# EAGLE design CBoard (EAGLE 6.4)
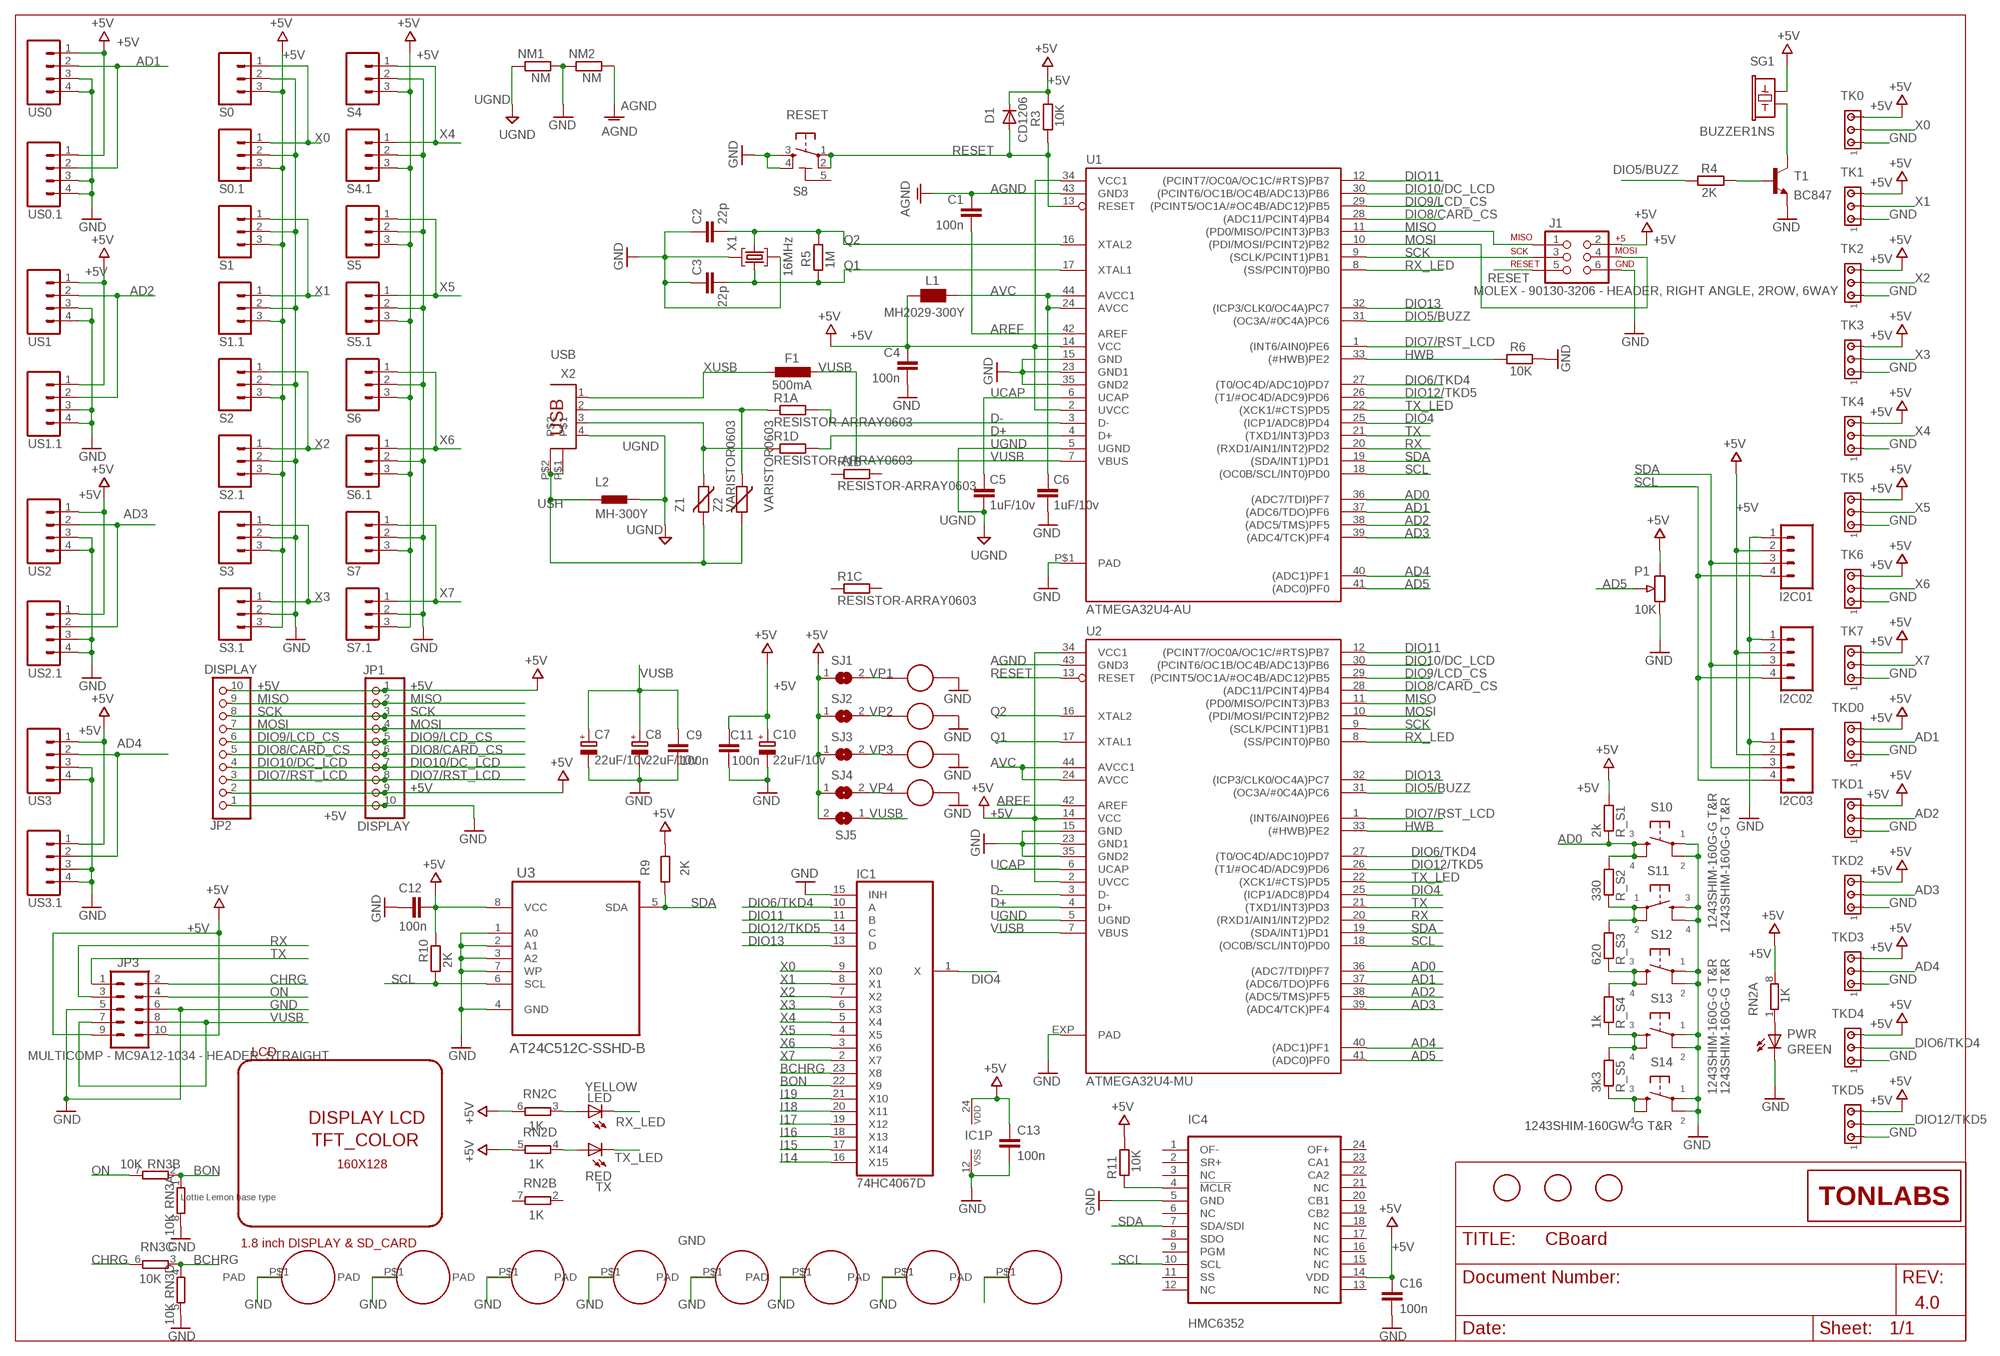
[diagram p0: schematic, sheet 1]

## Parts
1  FIDUCIALMOUNT  [FIDUCIA-MOUNT]
2  FIDUCIALMOUNT  [FIDUCIA-MOUNT]
3  FIDUCIALMOUNT  [FIDUCIA-MOUNT]
C1  100n  C-EUC0603  [C0603-ROUND]
C2  22p  C-EUC0603  [C0603-ROUND]
C3  22p  C-EUC0603  [C0603-ROUND]
C4  100n  C-EUC0603  [C0603-ROUND]
C5  1uF/10v  C-EUC0603  [C0603-ROUND]
C6  1uF/10v  C-EUC0603  [C0603-ROUND]
C7  22uF/10v  CPOL-EUSMCB  [SMC_B]
C8  22uF/10v  CPOL-EUSMCB  [SMC_B]
C9  100n  C-EUC0603  [C0603-ROUND]
C10  22uF/10v  CPOL-EUSMCB  [SMC_B]
C11  100n  C-EUC0603  [C0603-ROUND]
C12  100n  C-EUC0603  [C0603-ROUND]
C13  100n  C-EUC0603  [C0603-ROUND]
C16  100n  C-EUC0603  [C0603-ROUND]
D1  CD1206  DIODE-MINIMELF  [MINIMELF]
F1  500mA  L-EUL1812  [L1812]
G1  LOTTIE_LEMON_BASE_TYPE  [BASE_ROBOT_001]
H1  2.5-MOUNTING-HOLE  [2.5PAD]
H2  2.5-MOUNTING-HOLE  [2.5PAD]
H3  2.5-MOUNTING-HOLE  [2.5PAD]
H4  2.5-MOUNTING-HOLE  [2.5PAD]
H5  2.5-MOUNTING-HOLE  [2.5PAD]
H6  2.5-MOUNTING-HOLE  [2.5PAD]
H7  2.5-MOUNTING-HOLE  [2.5PAD]
H8  2.5-MOUNTING-HOLE  [2.5PAD]
I2C01  M04PTH  [1X04]
I2C02  M04PTH  [1X04]
I2C03  M04PTH  [1X04]
IC1  74HC4067D  4067D  [SO24W]
IC4  HMC6352  [HMC6352]
J1  MOLEX - 90130-3206 - HEADER, RIGHT ANGLE, 2ROW, 6WAY  AVR_SPI_PRG_6PTH  [2X3]
JP1  DISPLAY  PINHD-1X10TH  [1X10-TH]
JP2  DISPLAY  PINHD-1X10TH  [1X10-TH]
JP3  MULTICOMP - MC9A12-1034 - HEADER, STRAIGHT  M05X2SHD_LOCK  [2X5-SHROUDED_LOCK]
L1  MH2029-300Y  WE-CBF_0805  [0805]
L2  MH-300Y  BEAD0805  [BEAD-0805-SMT]
LCD  1.8 inch DISPLAY & SD_CARD  1.8-COLOR_TFT-LCD_DISPLAY_&_MICRO-SD  [1.8-LCD]
LED  YELLOW  LEDCHIP-LED0805  [CHIP-LED0805]
LOGO  LOGO-TONYLABSMED-LANDSCAPE  [LOGO-TONYLABS-MED-LANDSCAPE]
NM1  NM  R-EU_R0805  [R0805]
NM2  NM  R-EU_R0805  [R0805]
P1  10K  POT-VERTICAL  [POT-V]
PTZ1  LOTTIE_LEMON_PADS_SUP  [PADS_LOTTIE_LEMON_SUP]
PTZ2  LOTTIE_LEMON_PADS_SUP  [PADS_LOTTIE_LEMON_SUP]
PTZ3  LOTTIE_LEMON_PADS_SUP1  [PADS_LOTTIE_LEMON_SUP]
PTZ4  LOTTIE_LEMON_PADS_SUP1  [PADS_LOTTIE_LEMON_SUP]
PWR  LEDCHIP-LED0805  [CHIP-LED0805]
R1  RESISTOR-ARRAY0603  [RESISTOR-0603-SMT-ARRAY]
R3  10K  R-EU_R0603  [R0603-ROUND]
R4  2K  R-EU_R0603  [R0603-ROUND]
R5  1M  R-EU_R0603  [R0603-ROUND]
R6  10K  R-EU_R0603  [R0603-ROUND]
R9  2K  R-EU_R0603  [R0603-ROUND]
R10  2K  R-EU_R0603  [R0603-ROUND]
R11  10K  R-EU_R0603  [R0603-ROUND]
R_S1  2k  R-EU_R0603  [R0603-ROUND]
R_S2  330  R-EU_R0603  [R0603-ROUND]
R_S3  620  R-EU_R0603  [R0603-ROUND]
R_S4  1k  R-EU_R0603  [R0603-ROUND]
R_S5  3k3  R-EU_R0603  [R0603-ROUND]
RN2  1K  4R-NCAY16  [CAY16]
RN3  10K  4R-NCAY16  [CAY16]
S0  M03PTH  [1X03]
S0.1  M03PTH  [1X03]
S1  M03PTH  [1X03]
S1.1  M03PTH  [1X03]
S2  M03PTH  [1X03]
S2.1  M03PTH  [1X03]
S3  M03PTH  [1X03]
S3.1  M03PTH  [1X03]
S4  M03PTH  [1X03]
S4.1  M03PTH  [1X03]
S5  M03PTH  [1X03]
S5.1  M03PTH  [1X03]
S6  M03PTH  [1X03]
S6.1  M03PTH  [1X03]
S7  M03PTH  [1X03]
S7.1  M03PTH  [1X03]
S8  RESET  TS42  [TS42]
S10  1243SHIM-160G-G T&R  TACTILE_SWITCHTACTILE_SWITCH_SMD-12MM  [TACTILE-SMD-12MM]
S11  1243SHIM-160G-G T&R  TACTILE_SWITCHTACTILE_SWITCH_SMD-12MM  [TACTILE-SMD-12MM]
S12  1243SHIM-160G-G T&R  TACTILE_SWITCHTACTILE_SWITCH_SMD-12MM  [TACTILE-SMD-12MM]
S13  1243SHIM-160G-G T&R  TACTILE_SWITCHTACTILE_SWITCH_SMD-12MM  [TACTILE-SMD-12MM]
S14  1243SHIM-160GW-G T&R  TACTILE_SWITCHTACTILE_SWITCH_SMD-12MM  [TACTILE-SMD-12MM]
SG1  BUZZER1NS  [BUZZER-12MM-NS]
SJ1  SJ  [SJ]
SJ2  SJ  [SJ]
SJ3  SJ  [SJ]
SJ4  SJ  [SJ]
SJ5  SJL  [SJL]
T1  BC847  [SOT23]
TK0  MTA03-100  [10X03MTA]
TK1  MTA03-100  [10X03MTA]
TK2  MTA03-100  [10X03MTA]
TK3  MTA03-100  [10X03MTA]
TK4  MTA03-100  [10X03MTA]
TK5  MTA03-100  [10X03MTA]
TK6  MTA03-100  [10X03MTA]
TK7  MTA03-100  [10X03MTA]
TKD0  MTA03-100  [10X03MTA]
TKD1  MTA03-100  [10X03MTA]
TKD2  MTA03-100  [10X03MTA]
TKD3  MTA03-100  [10X03MTA]
TKD4  MTA03-100  [10X03MTA]
TKD5  MTA03-100  [10X03MTA]
TX  RED  LEDCHIP-LED0805  [CHIP-LED0805]
U1  ATMEGA32U4-AU  ATMEGA32U4-XUAU  [TQFP44-PAD]
U2  ATMEGA32U4-MU  ATMEGA32U4-XUMU  [QFN44ML7X7]
U3  AT24C512C-SSHD-B  AT24C128BN-SH-B  [SOIC127P600X175-8N]
US0  M04PTH  [1X04]
US0.1  M04PTH  [1X04]
US1  M04PTH  [1X04]
US1.1  M04PTH  [1X04]
US2  M04PTH  [1X04]
US2.1  M04PTH  [1X04]
US3  M04PTH  [1X04]
US3.1  M04PTH  [1X04]
X1  16MHz  CRYSTAL-3.2-2.5  [CRYSTAL-3.2-2.5]
X2  USB  PN61729  [PN61729]
Z1  VARISTOR0603  [VARISTOR-0603-SMT]
Z2  VARISTOR0603  [VARISTOR-0603-SMT]

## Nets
+5V: C4.1 C10.+ C11.1 C12.1 C13.1 C16.1 D1.C I2C01.2 I2C02.2 I2C03.2 IC1.24(VDD) IC4.14(VDD) J1.2 JP1.1 JP1.9 JP2.2 JP2.10 JP3.9 JP3.10 L1.2 P1.B R3.1 R9.2 R10.1 R11.1 R_S1.2 RN2.5 RN2.6 RN2.8 S0.1.3 S0.3 S1.1.3 S1.3 S2.1.3 S2.3 S3.1.3 S3.3 S4.1.3 S4.3 S5.1.3 S5.3 S6.1.3 S6.3 S7.1.3 S7.3 SG1.+ SJ1.1 SJ2.1 SJ3.1 SJ4.1 SJ5.2 TK0.3 TK1.3 TK2.3 TK3.3 TK4.3 TK5.3 TK6.3 TK7.3 TKD0.3 TKD1.3 TKD2.3 TKD3.3 TKD4.3 TKD5.3 U1.2(UVCC) U1.14(VCC) U1.34(VCC1) U2.2(UVCC) U2.14(VCC) U2.34(VCC1) U3.8(VCC) US0.1 US0.1.1 US1.1 US1.1.1 US2.1 US2.1.1 US3.1 US3.1.1
AD0: R_S1.1 R_S2.2 S10.P$3 S10.P$4 U1.36((ADC7/TDI)PF7) U2.36((ADC7/TDI)PF7)
AD1: TKD0.2 U1.37((ADC6/TDO)PF6) U2.37((ADC6/TDO)PF6) US0.1.2 US0.2
AD2: TKD1.2 U1.38((ADC5/TMS)PF5) U2.38((ADC5/TMS)PF5) US1.1.2 US1.2
AD3: TKD2.2 U1.39((ADC4/TCK)PF4) U2.39((ADC4/TCK)PF4) US2.1.2 US2.2
AD4: TKD3.2 U1.40((ADC1)PF1) U2.40((ADC1)PF1) US3.1.2 US3.2
AD5: P1.C U1.41((ADC0)PF0) U2.41((ADC0)PF0)
AGND: C1.1 NM2.1 U1.43(GND3) U2.43(GND3)
AREF: C1.2 U1.42(AREF) U2.42(AREF)
AVC: C6.1 L1.1 U1.24(AVCC) U1.44(AVCC1) U2.24(AVCC) U2.44(AVCC1)
BCHRG: IC1.23(X8) RN3.3 RN3.4
BON: IC1.22(X9) RN3.1 RN3.2
CHRG: JP3.2 RN3.6
D+: R1.5 U1.4(D+) U2.4(D+)
D-: R1.8 U1.3(D-) U2.3(D-)
DIO4: IC1.1(X) U1.25((ICP1/ADC8)PD4) U2.25((ICP1/ADC8)PD4)
DIO5/BUZZ: R4.2 U1.31((OC3A/#0C4A)PC6) U2.31((OC3A/#0C4A)PC6)
DIO6/TKD4: IC1.10(A) TKD4.2 U1.27((T0/OC4D/ADC10)PD7) U2.27((T0/OC4D/ADC10)PD7)
DIO7/RST_LCD: JP1.8 JP2.3 U1.1((INT6/AIN0)PE6) U2.1((INT6/AIN0)PE6)
DIO8/CARD_CS: JP1.6 JP2.5 U1.28((ADC11/PCINT4)PB4) U2.28((ADC11/PCINT4)PB4)
DIO9/LCD_CS: JP1.5 JP2.6 U1.29((PCINT5/OC1A/#OC4B/ADC12)PB5) U2.29((PCINT5/OC1A/#OC4B/ADC12)PB5)
DIO10/DC_LCD: JP1.7 JP2.4 U1.30((PCINT6/OC1B/OC4B/ADC13)PB6) U2.30((PCINT6/OC1B/OC4B/ADC13)PB6)
DIO11: IC1.11(B) U1.12((PCINT7/OC0A/OC1C/#RTS)PB7) U2.12((PCINT7/OC0A/OC1C/#RTS)PB7)
DIO12/TKD5: IC1.14(C) TKD5.2 U1.26((T1/#OC4D/ADC9)PD6) U2.26((T1/#OC4D/ADC9)PD6)
DIO13: IC1.13(D) U1.32((ICP3/CLK0/OC4A)PC7) U2.32((ICP3/CLK0/OC4A)PC7)
GND: C2.1 C3.1 C4.2 C6.2 C7.- C8.- C9.2 C10.- C11.2 C12.2 C13.2 C16.2 H1.P$1(PAD) H2.P$1(PAD) H3.P$1(PAD) H4.P$1(PAD) H5.P$1(PAD) H6.P$1(PAD) H7.P$1(PAD) H8.P$1(PAD) I2C01.1 I2C02.1 I2C03.1 IC1.12(VSS) IC1.15(INH) IC4.5(GND) J1.6 JP1.10 JP2.1 JP3.5 JP3.6 NM1.1 NM2.2 P1.A PTZ1.P$52 PTZ2.P$52 PTZ3.P$52 PTZ4.P$52 PWR.C R6.1 RN3.5 RN3.8 S0.1.2 S0.2 S1.1.2 S1.2 S2.1.2 S2.2 S3.1.2 S3.2 S4.1.2 S4.2 S5.1.2 S5.2 S6.1.2 S6.2 S7.1.2 S7.2 S8.3 S8.4 S10.P$1 S10.P$2 S11.P$3 S11.P$4 S12.P$1 S12.P$2 S13.P$1 S13.P$2 S14.P$1 S14.P$2 T1.2(E) TK0.1 TK1.1 TK2.1 TK3.1 TK4.1 TK5.1 TK6.1 TK7.1 TKD0.1 TKD1.1 TKD2.1 TKD3.1 TKD4.1 TKD5.1 U1.15(GND) U1.23(GND1) U1.35(GND2) U1.P$1(PAD) U2.15(GND) U2.23(GND1) U2.35(GND2) U2.EXP(PAD) U3.1(A0) U3.2(A1) U3.3(A2) U3.4(GND) U3.7(WP) US0.1.3 US0.1.4 US0.3 US0.4 US1.1.3 US1.1.4 US1.3 US1.4 US2.1.3 US2.1.4 US2.3 US2.4 US3.1.3 US3.1.4 US3.3 US3.4 X1.2(GND) X1.4(GND)
HWB: R6.2 U1.33((#HWB)PE2) U2.33((#HWB)PE2)
I14: IC1.16(X15)
I15: IC1.17(X14)
I16: IC1.18(X13)
I17: IC1.19(X12)
I18: IC1.20(X11)
I19: IC1.21(X10)
MISO: J1.1 JP1.2 JP2.9 U1.11((PD0/MISO/PCINT3)PB3) U2.11((PD0/MISO/PCINT3)PB3)
MOSI: J1.4 JP1.4 JP2.7 U1.10((PDI/MOSI/PCINT2)PB2) U2.10((PDI/MOSI/PCINT2)PB2)
N$2: R1.1 X2.2 Z2.1
N$3: R1.4 X2.3 Z1.1
N$4: RN2.4 TX.A
N$5: IC4.4(!MCLR) R11.2
N$13: R_S2.1 R_S3.2 S11.P$1 S11.P$2
N$14: LED.A RN2.3
N$17: SG1.- T1.3(C)
N$24: PWR.A RN2.1
N$27: R_S3.1 R_S4.2 S12.P$3 S12.P$4
N$29: R_S4.1 R_S5.2 S13.P$3 S13.P$4
N$30: R_S5.1 S14.P$3 S14.P$4
N$31: R4.1 T1.1(B)
ON: JP3.4 RN3.7
Q1: C3.2 R5.2 U1.17(XTAL1) U2.17(XTAL1) X1.1(C1)
Q2: C2.2 R5.1 U1.16(XTAL2) U2.16(XTAL2) X1.3(C2)
RESET: D1.A J1.5 R3.2 S8.1 S8.2 U1.13(RESET) U2.13(RESET)
RX: JP3.3 U1.20((RXD1/AIN1/INT2)PD2) U2.20((RXD1/AIN1/INT2)PD2)
RX_LED: LED.C U1.8((SS/PCINT0)PB0) U2.8((SS/PCINT0)PB0)
SCK: J1.3 JP1.3 JP2.8 U1.9((SCLK/PCINT1)PB1) U2.9((SCLK/PCINT1)PB1)
SCL: I2C01.4 I2C02.4 I2C03.4 IC4.10(SCL) R10.2 U1.18((OC0B/SCL/INT0)PD0) U2.18((OC0B/SCL/INT0)PD0) U3.6(SCL)
SDA: I2C01.3 I2C02.3 I2C03.3 IC4.7(SDA/SDI) R9.1 U1.19((SDA/INT1)PD1) U2.19((SDA/INT1)PD1) U3.5(SDA)
TX: JP3.1 U1.21((TXD1/INT3)PD3) U2.21((TXD1/INT3)PD3)
TX_LED: TX.C U1.22((XCK1/#CTS)PD5) U2.22((XCK1/#CTS)PD5)
UCAP: C5.1 U1.6(UCAP) U2.6(UCAP)
UGND: C5.2 L2.2 NM1.2 U1.5(UGND) U2.5(UGND) X2.4
USH: L2.1 X2.P$1 X2.P$2 Z1.2 Z2.2
VP1: PTZ3.P$42 SJ1.2
VP2: PTZ4.P$42 SJ2.2
VP3: PTZ1.P$42 SJ3.2
VP4: PTZ2.P$42 SJ4.2
VUSB: C7.+ C8.+ C9.1 F1.2 JP3.7 JP3.8 SJ5.1 U1.7(VBUS) U2.7(VBUS)
X0: IC1.9(X0) S0.1 S0.1.1 TK0.2
X1: IC1.8(X1) S1.1 S1.1.1 TK1.2
X2: IC1.7(X2) S2.1 S2.1.1 TK2.2
X3: IC1.6(X3) S3.1 S3.1.1 TK3.2
X4: IC1.5(X4) S4.1 S4.1.1 TK4.2
X5: IC1.4(X5) S5.1 S5.1.1 TK5.2
X6: IC1.3(X6) S6.1 S6.1.1 TK6.2
X7: IC1.2(X7) S7.1 S7.1.1 TK7.2
XUSB: F1.1 X2.1
Unconnected: IC4.1(OF-) IC4.2(SR+) IC4.3(NC) IC4.6(NC) IC4.8(SDO) IC4.9(PGM) IC4.11(SS) IC4.12(NC) IC4.13(NC) IC4.15(NC) IC4.16(NC) IC4.17(NC) IC4.18(NC) IC4.19(CB2) IC4.20(CB1) IC4.21(NC) IC4.22(CA2) IC4.23(CA1) IC4.24(OF+) R1.2 R1.3 R1.6 R1.7 RN2.2 RN2.7

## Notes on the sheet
- GREEN
- 4.0

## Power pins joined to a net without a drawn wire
5-GND: S8.5(5-GND)

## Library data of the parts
1-3 = Smartprj:FIDUCIALMOUNT
C1-C6 C9 C11-C13 C16 = Smartprj:C-EU: CAPACITOR, European symbol
C7 C8 C10 = Smartprj:CPOL-EU: POLARIZED CAPACITOR, European symbol
D1 = diode:DIODE-: DIODE
F1 = rcl:L-EU: INDUCTOR, European symbol
G1 = complubot:LOTTIE_LEMON_BASE_TYPE: Lottie Lemon Robot Base
H1-H8 = tinker_it:2.5-MOUNTING-HOLE
I2C01-I2C03 US0 US0.1 US1 US1.1 US2 US2.1 US3 US3.1 = sparkfun:M04: Header 4 Standard 4-pin 0.1" header. Use with straight break away headers (SKU : PRT-00116), right angle break away headers (PRT-00553), swiss pins (PRT-00743), machine pins (PRT-00117), and female headers (PRT-00115). Molex polarized connector foot print use with SKU : PRT-08231 with associated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
IC1 = 40xx:4067: 16-channel ANALOG MULTIPLEXER
IC4 = Smartprj:HMC6352: HMC6352 2-Axis Compass with Algorithms Honeywell
J1 = sparkfun:AVR_SPI_PRG_6: AVR ISP 6 Pin This is the reduced ISP connector for AVR programming. Common on Arduino. This footprint will take up less PCB space and can be used with a 10-pin to 6-pin adapter such as SKU: BOB-08508
JP1 JP2 = Smartprj:PINHD-1X10: PIN HEADER
JP3 = Smartprj:M05X2: Header 5x2 Standard 10-pin dual row 0.1" header. Commonly used with AVR-ISP. Use with Spark Fun Electronics SKU: PRT-00778
L1 = wuerth-elektronik:WE-CBF: SMD EMI Suppression Ferrite Beads
L2 = TONYLABS:BEAD
LCD = Smartprj:1.8-COLOR_TFT-LCD_DISPLAY_&_MICRO-SD: 1.8 inch LCD_COLOR
LED PWR TX = led:LED: LED
LOGO = TONYLABS:LOGO-TONYLABS
NM1 NM2 = resistor:R-EU_: RESISTOR, European symbol
P1 = Smartprj:POT-VERTICAL: Vertical POT TinkerKit
PTZ1 PTZ2 = Lottie_SPad2:LOTTIE_LEMON_PADS_SUP
PTZ3 PTZ4 = Lottie_SPad:LOTTIE_LEMON_PADS_SUP1
R1 = TONYLABS:RESISTOR-ARRAY; PACKAGE: 0603
R3-R6 R9-R11 R_S1-R_S5 = Smartprj:R-EU_: RESISTOR, European symbol
RN2 RN3 = resistor-dil:4R-N: Array Chip Resistor Source: RS Component / Phycomp; OC_FARNELL: unknown; OC_NEWARK: unknown
S0 S0.1 S1 S1.1 S2 S2.1 S3 S3.1 S4 S4.1 S5 S5.1 S6 S6.1 S7 S7.1 = sparkfun:M03: Header 3 Standard 3-pin 0.1" header. Use with straight break away headers (SKU : PRT-00116), right angle break away headers (PRT-00553), swiss pins (PRT-00743), machine pins (PRT-00117), and female headers (PRT-00115). Molex polarized connector foot print use with SKU : PRT-08232 with associated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
S8 = Smartprj:TS42: TS42 Dongnan Electronics Tact switch VDC 12V - 50mA
S10-S14 = Smartprj:TACTILE_SWITCH: Momentary Switch Button commonly used for reset or general input.
SG1 = Smartprj:BUZZER1: Buzzer 12-22mm
SJ1-SJ5 = Smartprj:SJ: SMD solder JUMPER
T1 = transistor:BC847: NPN TRANSISTOR
TK0 TK1-TK7 TKD0 TKD1-TKD5 = con-amp:MTA03-100: AMP connector
U1 U2 = Smartprj:ATMEGA32U4-XU
U3 = Smartprj:AT24C128BN-SH-B: Two-wire Serial EEPROM; MPN: AT24C128BN-SH-B; OC_FARNELL: 1362649; OC_NEWARK: 50M3322; PACKAGE: SOIC-8; SUPPLIER: Atmel
X1 = Smartprj:CRYSTAL-3.2-2.5
X2 = Smartprj:PN61729: BERG USB connector
Z1 Z2 = TONYLABS:VARISTOR: Varistor

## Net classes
0 default: width 0.254 mm, drill 0.584 mm, clearance 0.178 mm
1 +5V: width 0.254 mm, drill 0.787 mm, clearance 0.178 mm
2 gnd: width 0.254 mm, drill 0.584 mm, clearance 0.178 mm

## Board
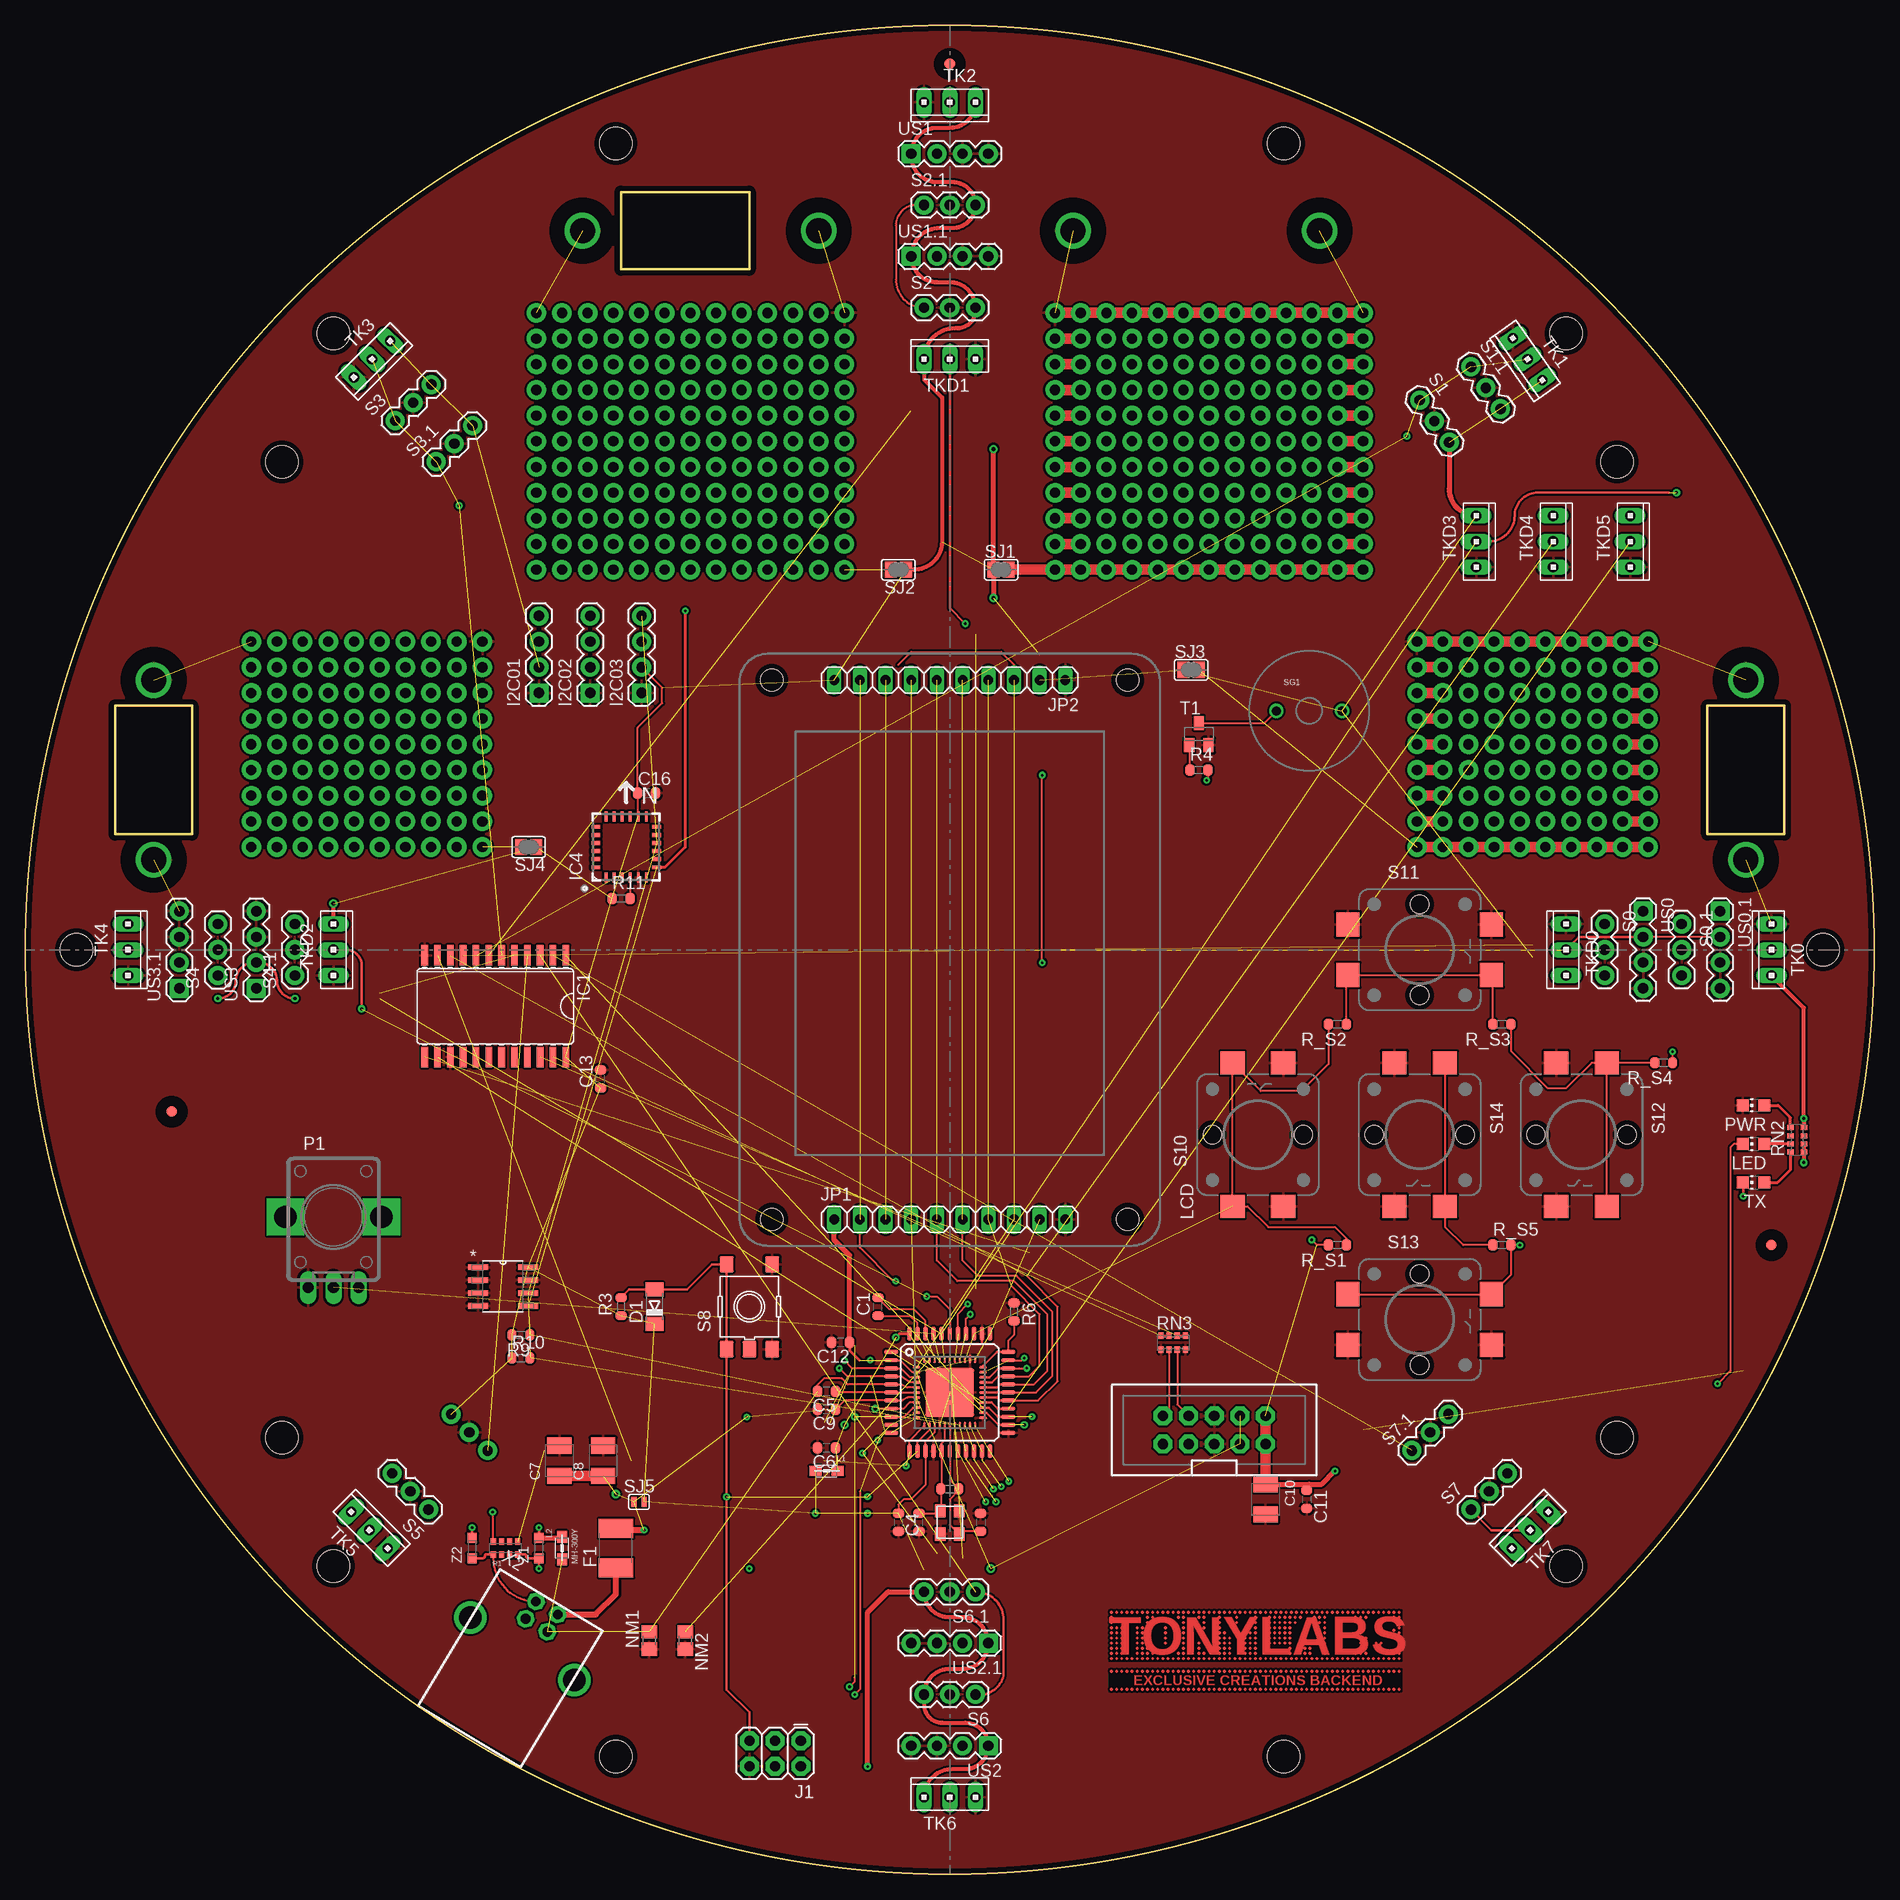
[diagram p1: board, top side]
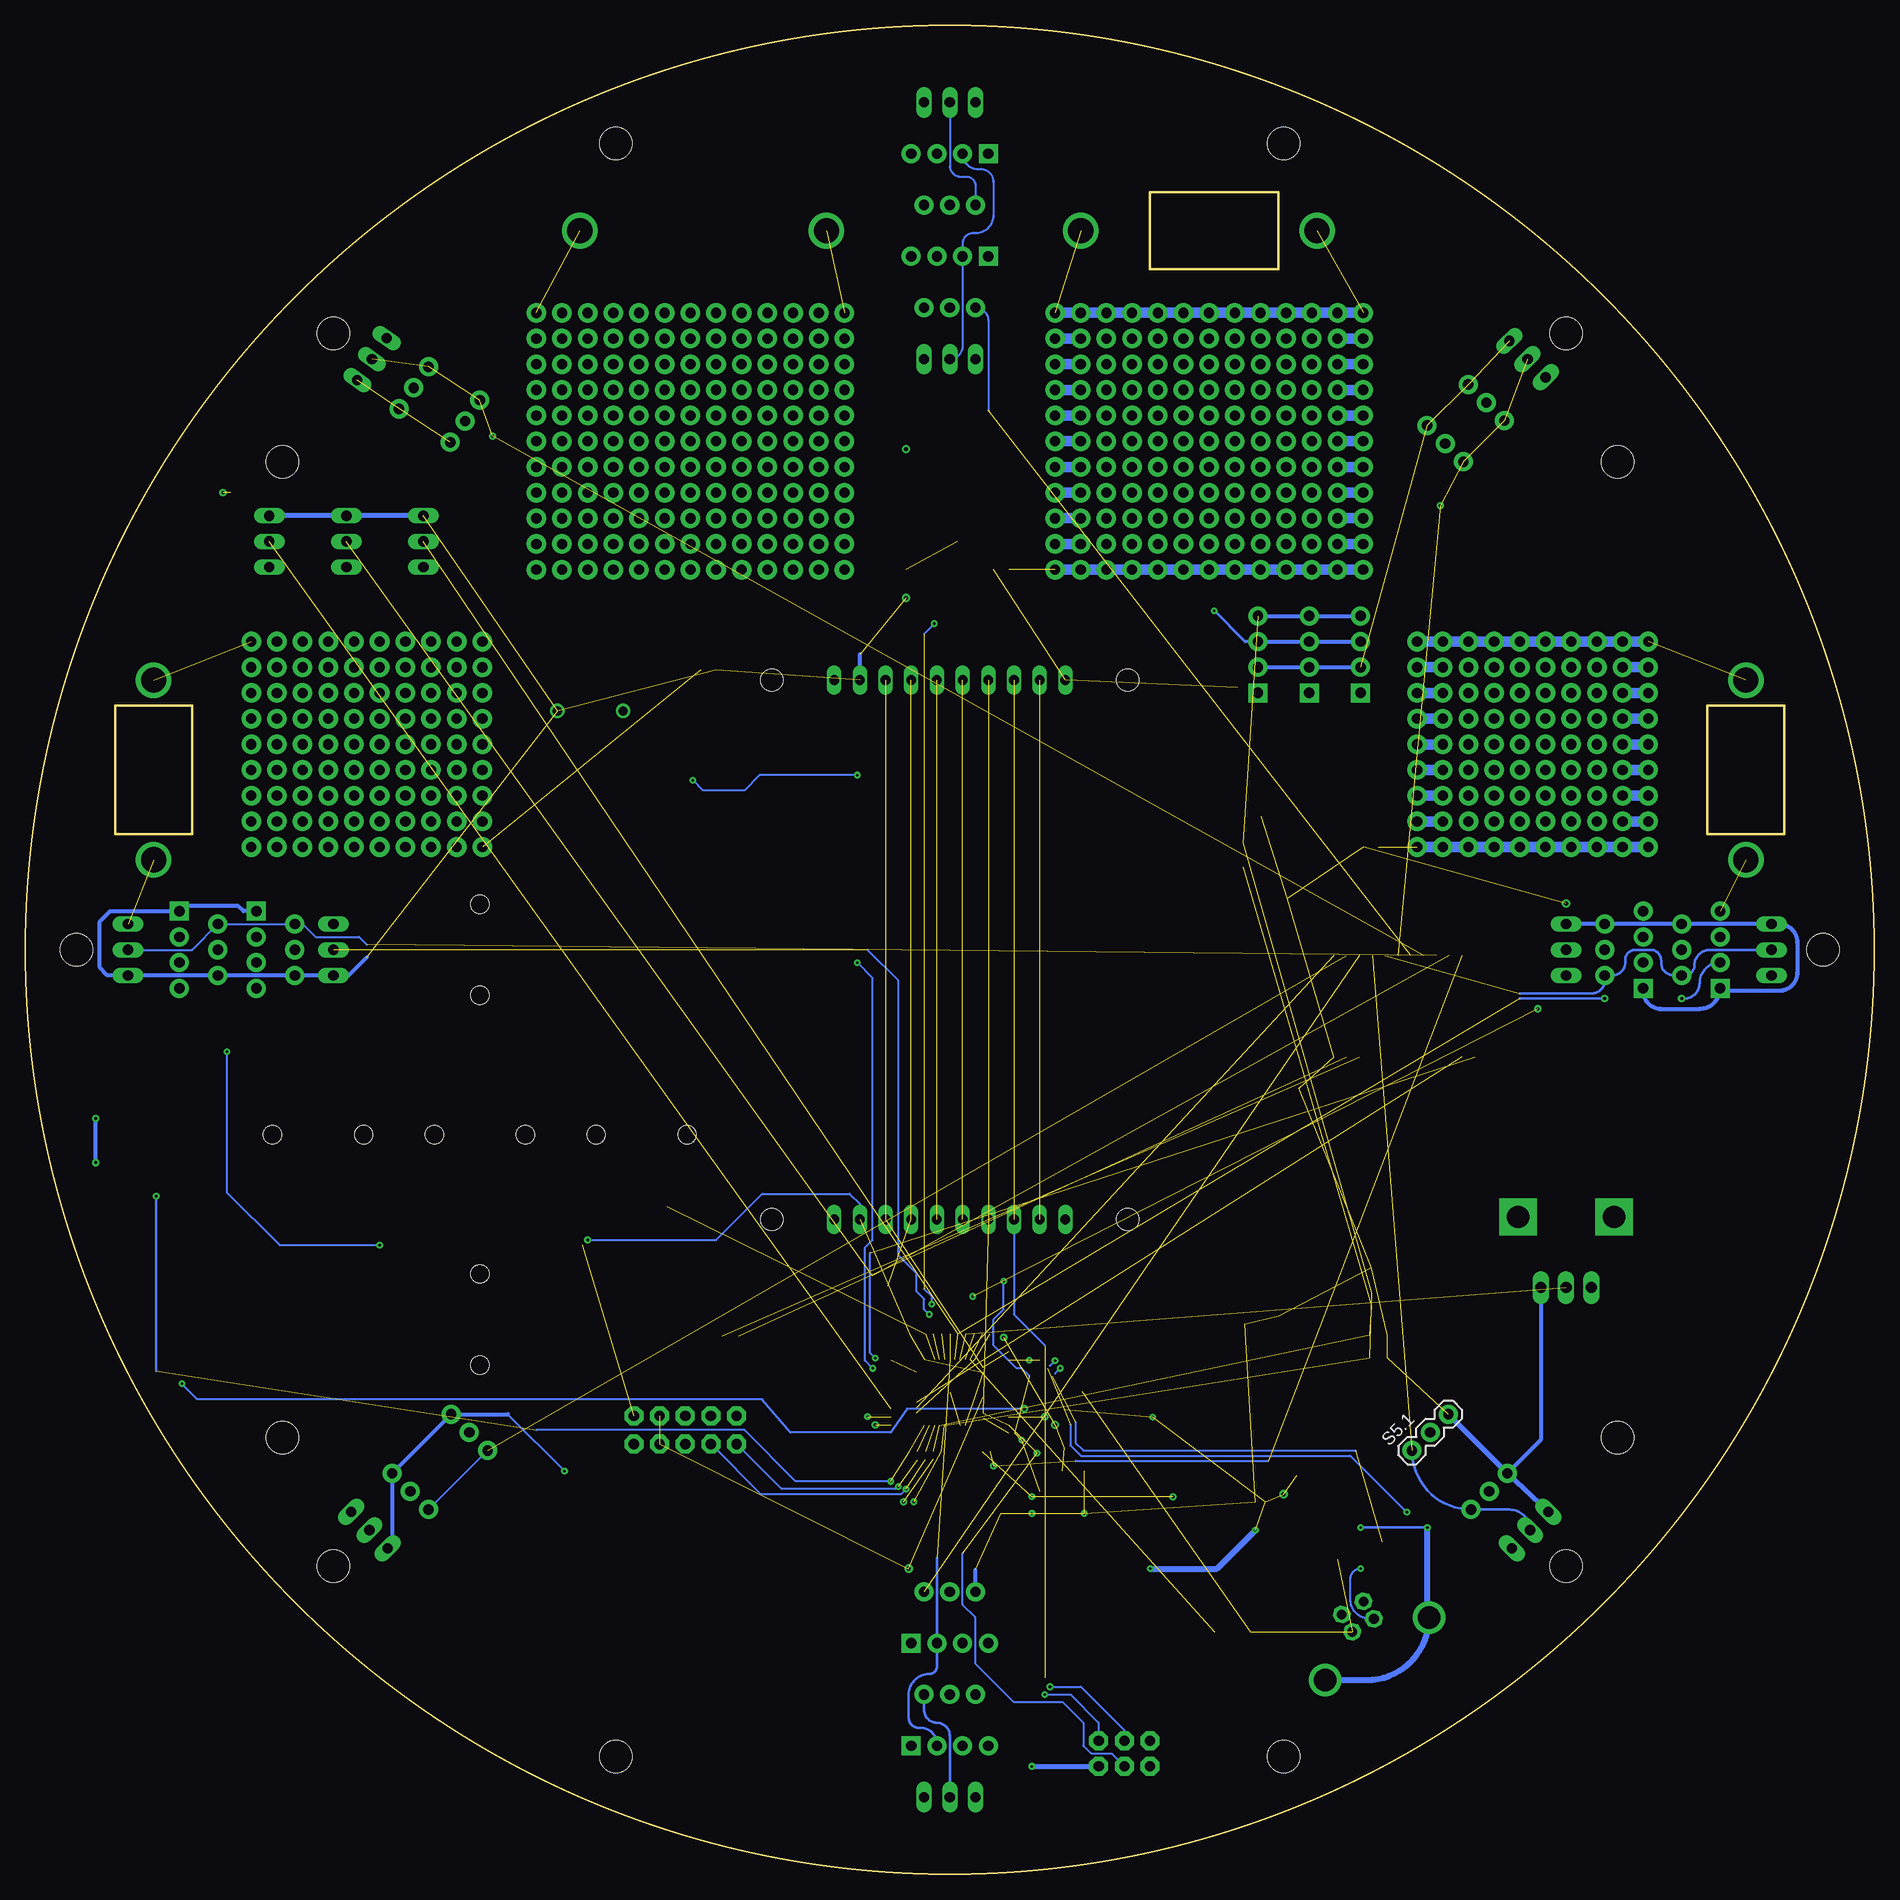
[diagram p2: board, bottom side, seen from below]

Size 182.88 x 182.88 mm. Coordinates in mm from the lower left corner, seen from the top.
Outline: 8.89,115.57 16.51,115.57 16.51,102.87 8.89,102.87 8.89,115.57
Outline: 166.37,115.57 173.99,115.57 173.99,102.87 166.37,102.87 166.37,115.57
Outline: 58.93,158.75 58.93,166.37 71.63,166.37 71.63,158.75 58.93,158.75
Copper layers (1*16): Top 0.035mm / dielectric 1.5mm / Bottom 0.035mm
Design rules "default *": minimum track width 10mil, minimum drill 24mil, track to track 8mil, track to pad 8mil, pad to pad 8mil, via to via 8mil, smd to smd 8mil, copper to edge 20mil, drill to drill 8mil, minimum pad ring 10mil, minimum via ring 8mil, stop-mask expansion 4mil, vias tented up to drill 0mil, thermal gap 10mil

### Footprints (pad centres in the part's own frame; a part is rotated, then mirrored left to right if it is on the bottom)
FIDUCIA-MOUNT = smd 1.016 x 1.016: P$1 0,0
C0603-ROUND = smd 0.898 x 1.1: 1 -0.889,0; 2 0.889,0
SMC_B = smd 1.6 x 2.4: + -1.5,0; - 1.5,0
MINIMELF = smd 1.4 x 1.8: A 1.7,0; C -1.7,0
L1812 = smd 1.9 x 3.4: 1 -1.95,0; 2 1.95,0
BASE_ROBOT_001 = hole 3.2: 5.08,91.44; 152.4,152.4; 30.48,152.4; 177.8,91.44; 30.48,30.48; 152.4,30.48; 58.42,171.196; 124.46,171.196; 58.42,11.659; 124.46,11.659; 25.375,139.7; 25.375,43.18; 157.455,139.7; 157.455,43.18
2.5PAD = drill 2.5 pad 3.5: P$1 0,0
1X04 = drill 1.016 pad 1.88 square: 1 0,0 | drill 1.016 pad 1.88: 2 2.54,0; 3 5.08,0; 4 7.62,0
SO24W = smd 0.66 x 2.032: 1 -6.985,-5.029; 2 -5.715,-5.029; 3 -4.445,-5.029; 4 -3.175,-5.029; 5 -1.905,-5.029; 6 -0.635,-5.029; 7 0.635,-5.029; 8 1.905,-5.029; 9 3.175,-5.029; 10 4.445,-5.029; 11 5.715,-5.029; 12 6.985,-5.029; 13 6.985,5.029; 14 5.715,5.029; 15 4.445,5.029; 16 3.175,5.029; 17 1.905,5.029; 18 0.635,5.029; 19 -0.635,5.029; 20 -1.905,5.029; 21 -3.175,5.029; 22 -4.445,5.029; 23 -5.715,5.029; 24 -6.985,5.029
HMC6352 = smd 1 x 0.4: 1 -3,2; 2 -3,1.2; 3 -3,0.4; 4 -3,-0.4; 5 -3,-1.2; 6 -3,-2; 13 3,-2; 14 3,-1.2; 15 3,-0.4; 16 3,0.4; 17 3,1.2; 18 3,2 | smd 0.4 x 1: 7 -2,-3; 8 -1.2,-3; 9 -0.4,-3; 10 0.4,-3; 11 1.2,-3; 12 2,-3; 19 2,3; 20 1.2,3; 21 0.4,3; 22 -0.4,3; 23 -1.2,3; 24 -2,3
2X3 = drill 1.016 pad 1.88 octagon: 1 0,0; 2 0,2.54; 3 2.54,0; 4 2.54,2.54; 5 5.08,0; 6 5.08,2.54
1X10-TH = drill 0.95 pad 1.422 long: 1 -11.43,0; 2 -8.89,0; 3 -6.35,0; 4 -3.81,0; 5 -1.27,0; 6 1.27,0; 7 3.81,0; 8 6.35,0; 9 8.89,0; 10 11.43,0
2X5-SHROUDED_LOCK = drill 1.016 pad 1.88 octagon: 1 -1.397,5.08; 2 1.397,5.08; 3 -1.397,2.54; 4 1.397,2.54; 5 -1.397,0; 6 1.397,0; 7 -1.397,-2.54; 8 1.397,-2.54; 9 -1.397,-5.08; 10 1.397,-5.08
0805 = smd 1.2 x 1: 1 -1.1,0; 2 1.1,0
BEAD-0805-SMT = smd 1.2 x 1: 1 -1.1,0; 2 1.1,0
1.8-LCD = hole 2.2: -26.67,17.607; -26.67,-17.607; 26.67,17.607; 26.67,-17.607
CHIP-LED0805 = smd 1.2 x 1.2: A 0,-1.05; C 0,1.05
R0805 = smd 1.3 x 1.5: 1 -0.85,0; 2 0.85,0
POT-V = drill 1.1 long: A -2.5,-7; B 2.5,-7; C 0,-7 | drill 2.2 pad 3.683 square: P$4 4.75,0; P$5 -4.75,0
PADS_LOTTIE_LEMON_SUP = drill 1 pad 1.93: P$1 -2.54,-12.7; P$2 -2.54,-15.24; P$3 -2.54,-17.78; P$4 -2.54,-20.32; P$5 -2.54,-22.86; P$6 -2.54,-25.4; P$7 -2.54,-27.94; P$8 -5.08,-12.7; P$9 -5.08,-15.24; P$10 -5.08,-17.78; P$11 -5.08,-20.32; P$12 -5.08,-22.86; P$13 -5.08,-25.4; P$14 -5.08,-27.94; P$15 -7.62,-12.7; P$16 -7.62,-15.24; P$17 -7.62,-17.78; P$18 -7.62,-22.86; P$19 -7.62,-20.32; P$20 -7.62,-27.94; P$21 -7.62,-25.4; P$22 -10.16,-12.7; P$23 -10.16,-15.24; P$24 -10.16,-17.78; P$25 -10.16,-10.16; P$26 -12.7,-10.16; P$27 -15.24,-10.16; P$28 -17.78,-10.16; P$30 -20.32,-10.16; P$31 -20.32,-12.7; P$42 2.54,-7.62; P$46 2.54,-10.16; P$47 2.54,-12.7; P$48 2.54,-15.24; P$49 2.54,-17.78; P$50 2.54,-22.86; P$51 2.54,-20.32; P$52 2.54,-27.94; P$53 2.54,-25.4; P$55 0,-7.62; P$57 0,-10.16; P$58 0,-12.7; P$59 0,-15.24; P$60 0,-17.78; P$61 0,-20.32; P$62 0,-22.86; P$63 0,-25.4; P$64 0,-27.94; P$91 -10.16,-20.32; P$105 -10.16,-22.86; P$108 -2.54,-7.62; P$111 -2.54,-10.16; P$112 -10.16,-25.4; P$115 -5.08,-7.62; P$120 -7.62,-7.62; P$123 -10.16,-27.94; P$126 -10.16,-7.62; P$129 -12.7,-12.7; P$132 -12.7,-7.62; P$135 -12.7,-15.24; P$138 -15.24,-7.62; P$141 -12.7,-17.78; P$144 -17.78,-7.62; P$147 -12.7,-20.32; P$150 -20.32,-7.62; P$152 -12.7,-22.86; P$156 -5.08,-10.16; P$157 -7.62,-10.16; P$158 -12.7,-25.4; P$159 -12.7,-27.94; P$160 -15.24,-12.7; P$161 -15.24,-15.24; P$162 -15.24,-17.78; P$163 -15.24,-20.32; P$164 -15.24,-22.86; P$165 -15.24,-25.4; P$166 -15.24,-27.94; P$167 -17.78,-15.24; P$168 -17.78,-12.7; P$169 -17.78,-17.78; P$170 -17.78,-20.32; P$171 -17.78,-22.86; P$172 -17.78,-25.4; P$173 -17.78,-27.94; P$174 -20.32,-15.24; P$175 -20.32,-17.78; P$176 -20.32,-20.32; P$177 -20.32,-22.86; P$178 -20.32,-25.4; P$179 -20.32,-27.94
PADS_LOTTIE_LEMON_SUP' = drill 1 pad 1.93: P$1 -2.54,-12.7; P$2 -2.54,-15.24; P$3 -2.54,-17.78; P$4 -2.54,-20.32; P$5 -2.54,-22.86; P$6 -2.54,-25.4; P$7 -2.54,-27.94; P$8 -5.08,-12.7; P$9 -5.08,-15.24; P$10 -5.08,-17.78; P$11 -5.08,-20.32; P$12 -5.08,-22.86; P$13 -5.08,-25.4; P$14 -5.08,-27.94; P$15 -7.62,-12.7; P$16 -7.62,-15.24; P$17 -7.62,-17.78; P$18 -7.62,-22.86; P$19 -7.62,-20.32; P$20 -7.62,-27.94; P$21 -7.62,-25.4; P$22 -10.16,-12.7; P$23 -10.16,-15.24; P$24 -10.16,-17.78; P$25 -10.16,-10.16; P$26 -12.7,-10.16; P$27 -15.24,-10.16; P$28 -17.78,-10.16; P$29 -20.32,-7.62; P$30 -20.32,-10.16; P$31 -20.32,-12.7; P$42 10.16,-2.54; P$43 10.16,-5.08; P$44 7.62,-7.62; P$45 10.16,-7.62; P$46 10.16,-10.16; P$47 10.16,-12.7; P$48 10.16,-15.24; P$49 10.16,-17.78; P$50 10.16,-22.86; P$51 10.16,-20.32; P$52 10.16,-27.94; P$53 10.16,-25.4; P$55 7.62,-2.54; P$56 7.62,-5.08; P$57 7.62,-10.16; P$58 7.62,-12.7; P$59 7.62,-15.24; P$60 7.62,-17.78; P$61 7.62,-20.32; P$62 7.62,-22.86; P$63 7.62,-25.4; P$64 7.62,-27.94; P$67 5.08,-2.54; P$68 5.08,-5.08; P$69 5.08,-7.62; P$70 5.08,-10.16; P$71 5.08,-12.7; P$72 5.08,-15.24; P$73 5.08,-17.78; P$74 5.08,-20.32; P$75 5.08,-22.86; P$76 5.08,-25.4; P$77 5.08,-27.94; P$80 2.54,-2.54; P$81 2.54,-5.08; P$82 2.54,-7.62; P$83 2.54,-10.16; P$84 2.54,-12.7; P$85 2.54,-15.24; P$86 2.54,-17.78; P$87 2.54,-20.32; P$88 2.54,-22.86; P$89 2.54,-25.4; P$90 2.54,-27.94; P$91 -10.16,-20.32; P$94 0,-2.54; P$95 0,-5.08; P$96 0,-10.16; P$97 0,-7.62; P$98 0,-15.24; P$99 0,-12.7; P$100 0,-17.78; P$101 0,-20.32; P$102 0,-22.86; P$103 0,-25.4; P$104 0,-27.94; P$105 -10.16,-22.86; P$108 -2.54,-2.54; P$109 -2.54,-5.08; P$110 -2.54,-7.62; P$111 -2.54,-10.16; P$112 -10.16,-25.4; P$115 -5.08,-2.54; P$116 -5.08,-5.08; P$117 -5.08,-7.62; P$118 -7.62,-7.62; P$119 -7.62,-5.08; P$120 -7.62,-2.54; P$123 -10.16,-27.94; P$124 -10.16,-7.62; P$125 -10.16,-5.08; P$126 -10.16,-2.54; P$129 -12.7,-12.7; P$130 -12.7,-7.62; P$131 -12.7,-5.08; P$132 -12.7,-2.54; P$135 -12.7,-15.24; P$136 -15.24,-7.62; P$137 -15.24,-5.08; P$138 -15.24,-2.54; P$141 -12.7,-17.78; P$142 -17.78,-7.62; P$143 -17.78,-5.08; P$144 -17.78,-2.54; P$147 -12.7,-20.32; P$150 -20.32,-2.54; P$151 -20.32,-5.08; P$152 -12.7,-22.86; P$156 -5.08,-10.16; P$157 -7.62,-10.16; P$158 -12.7,-25.4; P$159 -12.7,-27.94; P$160 -15.24,-12.7; P$161 -15.24,-15.24; P$162 -15.24,-17.78; P$163 -15.24,-20.32; P$164 -15.24,-22.86; P$165 -15.24,-25.4; P$166 -15.24,-27.94; P$167 -17.78,-15.24; P$168 -17.78,-12.7; P$169 -17.78,-17.78; P$170 -17.78,-20.32; P$171 -17.78,-22.86; P$172 -17.78,-25.4; P$173 -17.78,-27.94; P$174 -20.32,-15.24; P$175 -20.32,-17.78; P$176 -20.32,-20.32; P$177 -20.32,-22.86; P$178 -20.32,-25.4; P$179 -20.32,-27.94
RESISTOR-0603-SMT-ARRAY = smd 0.5 x 0.65: 1 -1.2,-0.625; 2 -0.4,-0.625; 3 0.4,-0.625; 4 1.2,-0.625; 5 1.2,0.625; 6 0.4,0.625; 7 -0.4,0.625; 8 -1.2,0.625
R0603-ROUND = smd 0.898 x 1.1: 1 -0.889,0; 2 0.889,0
CAY16 = smd 0.5 x 0.65: 1 -1.2,-0.675; 2 -0.4,-0.675; 3 0.4,-0.675; 4 1.2,-0.675; 5 1.2,0.675; 6 0.4,0.675; 7 -0.4,0.675; 8 -1.2,0.675
1X03 = drill 1.016 pad 1.88: 1 0,0; 2 2.54,0; 3 5.08,0
TS42 = smd 1.6 x 1.4: 1 -4.2,2.25; 2 4.2,2.25; 3 -4.2,-2.25; 4 4.2,-2.25; 5 -4.2,0
TACTILE-SMD-12MM = smd 2.3 x 2.4: P$1 7.1,-2.5; P$2 -7.1,-2.5; P$3 7.1,2.5; P$4 -7.1,2.5 | hole 1.8: 0,4.5; 0,-4.5
BUZZER-12MM-NS = drill 0.9: + 3.25,0; - -3.25,0
SJ = smd 1.168 x 1.6: 1 -0.762,0; 2 0.762,0
SJL = smd 0.508 x 1.016: 1 -0.508,0; 2 0.508,0
SOT23 = smd 1 x 1.4: 1 -0.95,-1.1; 2 0.95,-1.1; 3 0,1.1
10X03MTA = drill 1.016 long: 1 2.54,0; 2 0,0; 3 -2.54,0
TQFP44-PAD = smd 1.4 x 0.45: 1 -5.8,4; 2 -5.8,3.2; 3 -5.8,2.4; 4 -5.8,1.6; 5 -5.8,0.8; 6 -5.8,0; 7 -5.8,-0.8; 8 -5.8,-1.6; 9 -5.8,-2.4; 10 -5.8,-3.2; 11 -5.8,-4; 23 5.8,-4; 24 5.8,-3.2; 25 5.8,-2.4; 26 5.8,-1.6; 27 5.8,-0.8; 28 5.8,0; 29 5.8,0.8; 30 5.8,1.6; 31 5.8,2.4; 32 5.8,3.2; 33 5.8,4 | smd 0.45 x 1.4: 12 -4,-5.8; 13 -3.2,-5.8; 14 -2.4,-5.8; 15 -1.6,-5.8; 16 -0.8,-5.8; 17 0,-5.8; 18 0.8,-5.8; 19 1.6,-5.8; 20 2.4,-5.8; 21 3.2,-5.8; 22 4,-5.8; 34 4,5.8; 35 3.2,5.8; 36 2.4,5.8; 37 1.6,5.8; 38 0.8,5.8; 39 0,5.8; 40 -0.8,5.8; 41 -1.6,5.8; 42 -2.4,5.8; 43 -3.2,5.8; 44 -4,5.8 | smd 1 x 1: P$1 0,0
QFN44ML7X7 = smd 0.75 x 0.275: 1 -3.275,2.5; 2 -3.275,2; 3 -3.275,1.5; 4 -3.275,1; 5 -3.275,0.5; 6 -3.275,0; 7 -3.275,-0.5; 8 -3.275,-1; 9 -3.275,-1.5; 10 -3.275,-2; 11 -3.275,-2.5; 23 3.275,-2.5; 24 3.275,-2; 25 3.275,-1.5; 26 3.275,-1; 27 3.275,-0.5; 28 3.275,0; 29 3.275,0.5; 30 3.275,1; 31 3.275,1.5; 32 3.275,2; 33 3.275,2.5 | smd 0.275 x 0.75: 12 -2.5,-3.275; 13 -2,-3.275; 14 -1.5,-3.275; 15 -1,-3.275; 16 -0.5,-3.275; 17 0,-3.275; 18 0.5,-3.275; 19 1,-3.275; 20 1.5,-3.275; 21 2,-3.275; 22 2.5,-3.275; 34 2.5,3.275; 35 2,3.275; 36 1.5,3.275; 37 1,3.275; 38 0.5,3.275; 39 0,3.275; 40 -0.5,3.275; 41 -1,3.275; 42 -1.5,3.275; 43 -2,3.275; 44 -2.5,3.275 | smd 4.826 x 4.826: EXP 0,0
SOIC127P600X175-8N = smd 1.981 x 0.559: 1 -2.464,1.905; 2 -2.464,0.635; 3 -2.464,-0.635; 4 -2.464,-1.905; 5 2.464,-1.905; 6 2.464,-0.635; 7 2.464,0.635; 8 2.464,1.905
CRYSTAL-3.2-2.5 = smd 1.3 x 1.05: 1 -1.15,-0.925; 2 1.15,-0.925; 3 1.15,0.925; 4 -1.15,0.925
PN61729 = drill 0.95 pad 1.676 octagon: 1 1.25,4.71; 2 -1.25,4.71; 3 -1.25,2.71; 4 1.25,2.71 | drill 2.2: P$1 -6,0; P$2 6,0
VARISTOR-0603-SMT = smd 1 x 1: 1 -1,0; 2 1,0

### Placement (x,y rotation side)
1  91.44,179.07 0 top
2  172.72,62.23 0 top
3  14.48,75.44 0 top
C1  84.33,56.13 90 top
C2  88.39,34.8 90 top
C3  94.49,34.8 270 top
C4  86.36,34.8 270 top
C5  79.25,47.75 180 top
C6  79.25,42.16 180 top
C7  52.83,40.89 90 top
C8  57.15,40.89 90 top
C9  79.25,45.97 180 top
C10  122.68,37.08 270 top
C11  126.75,37.08 270 top
C12  80.64,52.6 180 top
C13  56.9,78.66 90 top
C16  61.47,106.93 0 top
D1  62.23,56.13 90 top
F1  58.42,32.26 90 top
G1  0,0 0 top
H1  170.18,118.11 0 top
H2  78.49,162.56 0 top
H3  55.12,162.56 0 top
H4  12.7,118.11 0 top
H5  12.7,100.33 0 top
H6  128.02,162.56 0 top
H7  103.63,162.56 0 top
H8  170.18,100.33 0 top
I2C01  50.8,116.84 90 top
I2C02  55.88,116.84 90 top
I2C03  60.96,116.84 90 top
IC1  46.48,85.85 180 top
IC4  59.44,101.6 90 top
J1  76.71,13.21 180 top
JP1  91.44,64.77 0 top
JP2  91.44,118.11 180 top
JP3  117.6,43.94 90 top
L1  79.25,39.88 180 top
L2  53.09,32.26 270 top
LCD  91.44,91.44 90 top
LED  170.94,72.24 90 top
LOGO  121.67,22.1 0 top
NM1  61.72,23.11 90 top
NM2  65.28,23.11 270 top
P1  30.48,65.02 0 top
PTZ1  140.21,93.98 180 top
PTZ2  42.67,93.98 180 bottom
PTZ3  [PADS_LOTTIE_LEMON_SUP']  112.01,126.49 180 top
PTZ4  [PADS_LOTTIE_LEMON_SUP']  70.87,126.49 180 bottom
PWR  170.94,76.05 90 top
R1  47.5,32.26 0 top
R3  58.93,56.13 90 top
R4  116.08,109.22 0 top
R5  91.44,38.1 0 top
R6  97.79,55.63 270 top
R9  49.02,53.34 180 top
R10  49.02,51.05 0 top
R11  58.93,96.52 0 top
R_S1  129.79,62.23 180 top
R_S2  129.79,84.07 180 top
R_S3  146.05,84.07 180 top
R_S4  162.05,80.26 180 top
R_S5  146.05,62.23 0 top
RN2  175.26,72.64 270 top
RN3  113.54,52.58 180 top
S0  156.21,93.98 270 top
S0.1  163.83,93.98 270 top
S1  137.92,145.8 305 top
S1.1  143,149.1 305 top
S2  88.9,154.94 0 top
S2.1  88.9,165.1 0 top
S3  36.58,143.76 45 top
S3.1  40.64,139.7 45 top
S4  19.05,88.9 90 top
S4.1  26.67,88.9 90 top
S5  39.88,36.07 135 top
S5.1  45.72,41.91 45 bottom
S6  93.98,17.78 180 top
S6.1  93.98,27.94 180 top
S7  143,36.07 45 top
S7.1  137.16,41.91 45 top
S8  71.63,56.13 90 top
S10  121.92,73.15 90 top
S11  137.92,91.44 0 top
S12  153.92,73.15 270 top
S13  137.92,54.86 0 top
S14  137.92,73.15 270 top
SG1  127,115.06 0 top
SJ1  96.52,129.03 0 top
SJ2  86.36,129.03 180 top
SJ3  115.32,119.13 0 top
SJ4  49.78,101.6 180 top
SJ5  60.71,36.83 0 top
T1  116.08,112.78 0 top
TK0  172.72,91.44 90 top
TK1  148.59,149.86 125 top
TK2  91.44,175.26 180 top
TK3  34.29,149.86 225 top
TK4  10.16,91.44 270 top
TK5  34.04,34.04 315 top
TK6  91.44,7.62 0 top
TK7  148.84,34.04 45 top
TKD0  152.4,91.44 90 top
TKD1  91.44,149.86 0 top
TKD2  30.48,91.44 270 top
TKD3  143.51,131.83 270 top
TKD4  151.13,131.83 270 top
TKD5  158.75,131.83 270 top
TX  170.94,68.43 90 top
U1  91.44,47.65 0 top
U2  91.44,47.65 0 top
U3  47.25,58.12 0 top
US0  160.02,95.25 270 top
US0.1  167.64,95.25 270 top
US1  87.63,170.18 0 top
US1.1  87.63,160.02 0 top
US2  95.25,12.7 180 top
US2.1  95.25,22.86 180 top
US3  22.86,87.63 90 top
US3.1  15.24,87.63 90 top
X1  91.44,34.8 90 top
X2  49.16,22.3 329 top
Z1  50.8,32.26 90 top
Z2  44.2,32.26 90 top

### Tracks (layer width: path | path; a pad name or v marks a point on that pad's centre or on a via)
+5V  (via drill 0.25, 0.3, 0.41)  (37 unrouted)
  Top 0.203: C4.1 86.36,36.58 86.87,37.08 87.63,37.08 89.04,38.49 U1.14 89.04,42.81 89.94,43.71 U2.14 | R_S1.2 127.76,62.23 v127.25,62.74 | C13.1 56.84,77.78 | IC4.14 60.64,106.88 C16.1 60.58,113.41 62.99,115.82 62.99,117.35 I2C03.2 | C11.1 126.75,38.33 127,38.58 | U2.2 87.77,49.65 86.57,50.85 U1.2
  Top 0.305: C12.1 81.53,51.82 82.5,50.85
  Top 0.406: v175.92,70.38 175.94,70.4 RN2.5 RN2.6 | RN2.8 175.92,73.86 v175.92,74.75 175.92,85.7 TK0.3 | S6.1.3 arc90 91.44,25.4 92.71,25.4 arc-90 US2.1.1 arc-90 92.71,20.32 91.44,20.32 arc90 S6.3 88.9,16.76 arc90 90.68,14.99 92.96,14.99 arc-90 US2.1 arc-90 92.96,10.41 91.69,10.41 arc90 TK6.3 | TK2.3 arc-90 91.44,172.72 90.17,172.72 arc90 US1.1 87.63,169.93 arc90 90.17,167.39 91.69,167.39 arc-90 S2.1.3 arc-90 91.69,162.81 90.42,162.81 arc90 US1.1.1 arc90 90.17,157.48 91.44,157.48 arc-90 S2.3 93.98,154.69 arc-90 92.2,152.91 91.95,152.91 arc90 TKD1.3 88.9,147.83 90.68,146.05 90.68,131.83 arc-90 87.88,129.03 SJ2.1 | TKD2.3 v30.48,96.01
  Top 0.508: C10.+ 127,38.58 128.25,38.58 v129.54,39.88 | C12.1 81.53,61.22 80.01,62.74 JP1.1 | S1.3 140.84,137.04 arc90 TKD3.3 | v95.76,140.97 SJ1.1 v95.76,126.24 | v83.31,10.67 83.31,25.91 85.34,27.94 S6.1.3
  Top 1.016: JP3.10 JP3.9 C10.+
  Bottom 0.203: v127.25,62.74 114.55,62.74 109.98,67.31 101.35,67.31 100.33,66.29 JP1.9
  Bottom 0.254: 135.16,45.5 v129.54,39.88
  Bottom 0.406: I2C03.2 I2C02.2 I2C01.2 | JP2.2 100.33,120.65 | 149.1,90.68 150.88,88.9 TKD0.3 S0.3 S0.1.3 TK0.3 174.75,88.9 175.51,89.66 175.51,94.23 174.5,95.25 US0.1.1 167.13,95.76 161.8,95.76 161.29,95.25 US0.1 | TKD2.3 S4.1.3 S4.3 TK4.3 9.4,93.98 arc90 7.62,92.2 7.62,89.15 arc90 9.4,87.38 14.99,87.38 arc90 US3.1.1 arc90 17.27,85.6 21.08,85.6 arc90 22.86,87.38 US3.1 | v175.92,70.38 v175.92,74.75 | S6.1.3 88.9,30.1 | P1.B 32.98,42.97 S5.3 | TK7.3 146.59,32.69 S7.3 S7.1.3 135.16,45.5
  Bottom 0.508: TK5.3 S5.3 S5.1.3 | v83.31,10.67 J1.2 | TKD3.3 TKD4.3 TKD5.3
  other vias: 83.57,50.85 83.31,35.69 78.15,35.69
AD0  (2 unrouted)
  Top 0.203: R_S2.2 128.91,80.14 126.24,77.47 122.2,77.47 S10.P$3 S10.P$4 120.89,66.05 122.94,64.01 129.54,64.01 130.68,62.86 R_S1.1
AD1  (via drill 0.25)  (2 unrouted)
  Top 0.203: U1.37 93.04,54.94 v93.47,55.37 | US0.1.2 US0.2
  Top 0.254: US0.2 153.67,92.71 TKD0.2
  Bottom 0.203: v93.47,55.37 93.98,55.88 93.98,56.9 94.74,57.66 94.74,59.44 96.52,61.21 96.52,88.39 99.57,91.44
AD2  (via drill 0.25)  (2 unrouted)
  Top 0.203: U1.38 92.24,55.41 v93.22,56.39 | v92.96,123.7 91.44,125.22
  Top 0.254: 91.44,125.22 TKD1.2
  Bottom 0.203: v93.22,56.39 93.22,57.15 93.98,57.91 | 93.98,122.68 v92.96,123.7 | US1.2 arc-90 88.65,168.66 88.39,168.66 arc90 87.12,167.39 87.12,164.08 arc90 88.9,162.31 89.15,162.31 arc-90 90.17,161.29 US1.1.2 90.17,151.13 arc90 TKD1.2
AD3  (via drill 0.25, 0.3)  (3 unrouted)
  Top 0.203: v89.15,57.15 90.17,57.15 91.44,55.88 U1.39
  Top 0.254: TKD2.2 31.75,91.44 arc-90 33.27,89.92 v33.27,85.6
  Bottom 0.254: US2.2 arc-90 94.23,14.48 94.49,14.48 arc90 95.5,15.49 95.5,17.78 arc90 93.47,19.81 arc-90 92.71,20.57 US2.1.2 92.71,31.24
AD4  (via drill 0.3)  (4 unrouted)
  Top 0.254: v26.67,86.61 arc-90 24.89,88.39 arc90 23.11,90.17 US3.2 22.61,90.17 arc90 20.83,88.39 arc-90 v19.05,86.61 | TKD3.2 144.78,131.83 arc90 147.32,134.37 arc-90 149.61,136.65 162.56,136.65
  Bottom 0.254: v26.67,86.61 35.05,86.61 | v19.05,86.61 18.8,86.61 arc-90 17.27,88.14 arc90 US3.1.2
  other vias: 163.32,136.65
AD5  (2 unrouted)
AGND  (2 unrouted)
  Top 0.203: U1.43 88.24,54.51 87.5,55.24 C1.1
AREF  (1 unrouted)
  Top 0.203: U1.42 89.04,54.72 87.88,55.88 85.47,55.88 C1.2
AVC  (via drill 0.3, 0.41)  (6 unrouted)
  Top 0.254: U2.24 95.07,45.65 96.27,44.45 U1.24
  Top 0.305: U1.44 86.47,53.45 v86.11,53.09
  other vias: 81.03,44.45 98.81,44.45
BCHRG  (1 unrouted)
  Top 0.203: RN3.3 RN3.4
BON  (1 unrouted)
  Top 0.203: RN3.1 RN3.2
CHRG
  Top 0.203: RN3.6 113.14,45.95 JP3.2
D+  (via drill 0.25)  (2 unrouted)
  Top 0.203: v80.52,50.04 81.31,49.25 U1.4 86.64,49.25 87.5,48.65 U2.4
  Bottom 0.203: v80.52,50.04 81.03,49.53 | 78.99,44.7 78.99,42.67 78.23,41.91 51.31,41.91
D-  (via drill 0.25)  (1 unrouted)
  Top 0.203: v81.03,50.8 81.78,50.05 U1.3 86.6,50.05 87.5,49.15 U2.3 | v46.23,35.81 46.23,32.95 R1.8
  Bottom 0.203: v81.03,50.8 81.53,50.29 | 79.5,44.45 79.5,42.42 78.49,41.4 51.82,41.4 v46.23,35.81
DIO4  (via drill 0.25)  (2 unrouted)
  Top 0.254: U2.25 95.33,46.15 96.23,45.25 U1.25
  other vias: 99.57,45.25
DIO5/BUZZ  (via drill 0.25)
  Top 0.203: U1.31 98.31,50.05 v99.06,50.04 | v100.58,90.17 v100.58,108.71 | R4.2 116.97,108.33 v116.84,108.2
  Top 0.254: U2.31 95.38,49.15 96.28,50.05 U1.31
  Bottom 0.203: v100.58,90.17 99.06,88.65 99.06,62.74 99.82,61.98 99.82,50.8 v99.06,50.04 | v100.58,108.71 110.24,108.71 111.76,107.19 115.82,107.19 v116.84,108.2
DIO6/TKD4  (2 unrouted)
  Top 0.203: U1.27 100.19,46.85 102.11,48.77 102.11,56.13 99.06,59.18
  Top 0.254: U2.27 96.11,47.15 96.41,46.85 U1.27
DIO7/RST_LCD  (3 unrouted)
  Top 0.203: 86.36,119.63 87.63,120.9 96.52,120.9 97.79,119.63 JP2.3
DIO8/CARD_CS  (1 unrouted)
  Top 0.203: U1.28 99.97,47.65 101.6,49.28 101.6,55.63 98.04,59.18 94.23,59.18 92.71,60.71 JP1.6
  Top 0.254: U2.28 U1.28
DIO9/LCD_CS  (1 unrouted)
  Top 0.203: U1.29 99.76,48.45 101.09,49.78 101.09,55.37 97.79,58.67 92.2,58.67 90.17,60.71 JP1.5
  Top 0.254: U2.29 96.15,48.15 96.45,48.45 U1.29
DIO10/DC_LCD  (2 unrouted)
  Top 0.203: U1.30 99.29,49.25 100.33,50.29 100.33,55.37 97.54,58.17
  Top 0.254: U2.30 95.64,48.65 96.27,49.28 96.29,49.25 U1.30
DIO11  (via drill 0.25)  (3 unrouted)
  Top 0.203: U1.12 87.44,42.87 U2.12
  Top 0.254: U2.12 88.94,44.24
  Bottom 0.203: 78.99,40.89 59.94,40.89
  other vias: 87.12,40.39
DIO12/TKD5  (2 unrouted)
  Top 0.254: U2.26 95.59,46.65 96.19,46.05 U1.26
DIO13  (via drill 0.25)  (2 unrouted)
  Top 0.203: U1.32 98.6,50.85 v98.81,51.05
  Bottom 0.203: v98.81,51.05 99.31,51.56 99.31,61.47
GND  (9 unrouted)
  Top 0.254: U2.23 94.81,45.15 | U1.23 96.31,43.65 | U2.35 93.44,51.28 | U1.35 94.64,52.48
  pour Top: 91.44,183.13 183.13,183.13 183.13,3.56 183.13,1.27 183.13,-0.76 0,-0.76 0,180.59 0,181.86 0,182.88 0,183.13
HWB
  Top 0.203: U1.33 97.24,52.79 97.79,53.34 R6.2
  Top 0.254: U2.33 94.72,50.27 96.1,51.65 U1.33
MISO  (via drill 0.25)  (5 unrouted)
  Top 0.203: 82.55,37.85 82.55,18.29 v82.04,17.78 | U1.11 85.05,43.65 | v86.11,58.67 85.85,58.67 82.55,61.98 JP1.2
  Bottom 0.203: v82.04,17.78 79.5,17.78 76.71,14.99 J1.1 | 83.57,49.28 84.33,50.04 84.84,50.04 87.12,52.32 87.12,54.86 86.11,55.88 v86.11,58.67
  other vias: 84.33,42.93
MOSI  (via drill 0.25)  (5 unrouted)
  Top 0.305: U1.10
  Bottom 0.203: J1.4 75.44,11.94 77.47,11.94 78.23,12.7 78.23,14.99 80.26,17.02 85.09,17.02 88.9,20.83 88.9,25.4 90.17,26.67 90.17,31.75
  other vias: 82.8,41.66
N$2
  Top 0.203: R1.1 46.3,31.2 arc90 X2.2
  Top 0.254: Z2.1 45.23,31.26 arc90 45.47,31.5 arc-90 45.6,31.63 R1.1
N$3  (via drill 0.25)
  Top 0.203: v50.8,30.23 Z1.1
  Top 0.254: R1.4 49.39,31.63 arc-90 49.53,31.5 arc90 49.77,31.26 Z1.1
  Bottom 0.203: X2.3 49.91,25.27 arc90 51.82,27.18 51.82,29.21 arc90 v50.8,30.23
N$4
  Top 0.279: RN2.4 174.58,69.68 173.33,68.43 TX.A
N$5
  Top 0.203: IC4.4 59.84,96.54 R11.2
N$13
  Top 0.203: R_S3.2 145.16,88.8 S11.P$1 S11.P$2 130.68,88.8 R_S2.1
N$14
  Top 0.279: RN2.3 LED.A
N$17
  Top 0.203: T1.3 122.56,113.88 SG1.-
N$24
  Top 0.279: RN2.1 174.58,74.84 173.38,76.05 PWR.A
N$27
  Top 0.203: S12.P$3 S12.P$4 156.44,80.26 | R_S4.2 156.44,80.26 | 156.44,80.26 154.94,80.26 152.4,77.72 150.62,77.72 146.94,81.41 R_S3.1
N$29  (via drill 0.25)
  Top 0.203: S13.P$4 S13.P$3 146.94,59.28 R_S5.2 v147.83,62.23 | R_S4.1 v162.94,81.36
  Bottom 0.203: v162.94,81.36 162.94,67.44 157.73,62.23 v147.83,62.23
N$30
  Top 0.203: S14.P$4 S14.P$3 140.42,64.05 142.24,62.23 R_S5.1
N$31
  Top 0.203: T1.1 115.13,109.28 R4.1
ON
  Top 0.203: RN3.7 113.94,46.46 JP3.4
Q1
  Top 0.203: U2.17 U1.17 91.44,38.99 R5.2 92.33,37.97 91.44,37.08 91.44,34.57 X1.1 92.63,33.91 C3.2
Q2
  Top 0.203: C2.2 90.25,35.69 X1.3 90.55,35.98 R5.1 90.64,38.19 U1.16 90.64,42.63 90.94,42.93 U2.16
RESET  (via drill 0.25, 0.3)  (2 unrouted)
  Top 0.203: U2.13 89.44,43.97 88.24,42.77 U1.13
  Top 0.254: R3.2 59.74,57.83 D1.A 65.45,57.83 67.95,60.33 S8.2 S8.1 v69.38,37.35 v69.37,37.34 69.38,37.33 69.38,18.25 71.63,16 J1.5
  other vias: 83.31,37.34
RX  (via drill 0.25)  (2 unrouted)
  Top 0.203: U1.20 93.84,41.03
  Bottom 0.203: JP3.3 110.11,37.59 96.27,37.59 v95.76,38.1
RX_LED  (via drill 0.25, 0.3)
  Top 0.203: LED.C 169.01,72.24 168.66,71.88 168.66,49.78 v167.39,48.51 | v84.07,46.05 U1.8 86.87,46.05 87.47,46.65 U2.8
  Bottom 0.203: v167.39,48.51 165.86,46.99 109.98,46.99 107.19,43.69 97.28,43.69 95.68,46.05 v84.07,46.05
SCK  (via drill 0.3)  (4 unrouted)
  Top 0.203: U1.9 86.9,45.25 87.8,46.15 U2.9 | 82.02,19.43 82.02,19.02 v81.53,18.54
  Bottom 0.203: v81.53,18.54 78.49,18.54 74.17,14.22 J1.3 | JP1.3 85.09,55.37 82.04,52.32
  other vias: 82.04,45.25
SCL  (via drill 0.25)  (6 unrouted)
  Bottom 0.406: I2C03.4 I2C02.4 I2C01.4
  other vias: 95,36.83
SDA  (via drill 0.25)  (5 unrouted)
  Top 0.203: U1.19 93.04,41.07
  Top 0.279: v65.28,124.97 65.28,101.6 63.28,99.6 IC4.7
  Bottom 0.279: I2C03.3 62.23,121.92 v65.28,124.97
  Bottom 0.406: I2C03.3 I2C02.3 I2C01.3
  other vias: 96.01,36.83
TX  (via drill 0.25)  (2 unrouted)
  Top 0.203: U1.21 94.64,41
  Bottom 0.203: v96.52,38.35 96.77,38.1 108.08,38.1 JP3.1
TX_LED  (via drill 0.25)  (3 unrouted)
  Top 0.254: v169.93,67.06 169.93,68.39 TX.C
  Bottom 0.203: 132.33,43.94 111.76,43.94 106.68,38.86 v97.28,38.86
  Bottom 0.254: 169.93,49.78 v169.93,67.06
UCAP
  Top 0.203: C5.1 80.24,47.65 U1.6 U2.6
UGND  (3 unrouted)
  Top 0.203: C5.2 78.36,48.39 78.99,49.02 80.77,49.02 81.35,48.45 U1.5 86.68,48.45 87.23,48.15 U2.5
USH  (via drill 0.25)
  Top 0.254: Z2.2 v44.2,34.29 | v50.8,34.29 Z1.2
  Top 0.508: Z1.2 52.99,33.26 L2.1
  Bottom 0.254: v44.2,34.29 v50.8,34.29
  Bottom 0.61: X2.P$2 50.2,19.21 arc-90 X2.P$1 44.02,25.73 44.2,25.91 v44.2,34.29
VP1
  Top 1.016: PTZ3.P$42 SJ1.2
VP2  (1 unrouted)
VP3  (1 unrouted)
VP4  (1 unrouted)
VUSB  (via drill 0.25, 0.41)  (8 unrouted)
  Top 0.203: C9.1 81.01,46.85 U1.7 86.73,46.85 87.28,47.15 U2.7
  Top 0.61: v61.21,34.04 58.59,34.04 F1.2
  Top 1.016: C7.+ C8.+
  Bottom 0.61: v71.63,30.23 65.02,30.23 v61.21,34.04
  other vias: 58.42,37.59 95.5,30.23 71.37,45.21
X0  (1 unrouted)
  Bottom 0.203: TK0.2 166.37,91.44 S0.1.1 S0.1 | 155.45,93.98 154.18,92.71 149.86,92.71 149.1,91.95
  Bottom 0.254: S0.1 155.45,93.98
X1  (via drill 0.3)  (4 unrouted)
  other vias: 136.65,142.24
X2  (1 unrouted)
  Top 0.203: S2.1.1 88.14,165.1 arc90 86.11,163.07 86.11,157.73 arc90 S2.1
  Bottom 0.203: TK2.2 91.44,168.91 arc-90 90.17,167.89 89.92,167.89 arc90 88.9,167.13 S2.1.1 | S2.1 arc90 87.63,153.67 87.63,144.78
X3  (via drill 0.3)  (4 unrouted)
  other vias: 42.93,135.38
X4  (1 unrouted)
  Bottom 0.254: TK4.2 16.26,91.44 arc-90 17.78,89.92 arc90 18.8,88.9 S4.1 19.81,88.9 arc90 21.08,90.17 21.08,90.42 arc-90 22.1,91.44 23.62,91.44 arc-90 24.64,90.42 24.64,90.17 arc90 25.91,88.9 S4.1.1 26.67,88.39 arc90 27.94,87.12 35.05,87.12
X5  (1 unrouted)
  Bottom 0.254: TK5.2 arc-90 36.07,36.07 S5.1 arc90 S5.1.1
X6  (1 unrouted)
  Top 0.254: S6.1 94.49,17.78 arc90 96.77,20.07 96.77,25.15 arc90 S6.1.1
  Bottom 0.254: TK6.2 91.44,13.72 arc-90 92.71,14.99 arc90 93.98,16.26 S6.1
X7  (1 unrouted)
  Top 0.254: TK7.2 145.03,34.04 S7.1
  Bottom 0.254: S7.1 S7.1.1
XUSB
  Top 0.61: X2.1 56.43,25.69 58.42,27.69 F1.1

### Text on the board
tSilk: TKD1 | TKD1 | PWR | LED1 | TX | TKD6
